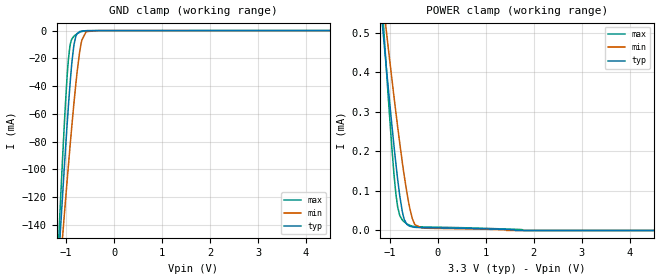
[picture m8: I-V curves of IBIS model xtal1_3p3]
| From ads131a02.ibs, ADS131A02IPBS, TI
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|   xtal1_3p3 Model
[Model]   xtal1_3p3
Model_type   Input
Vinl = 0.66
Vinh = 2.64
|   typ   min   max
|   (nom PVT)   (fast PVT)   (slow PVT)
C_comp   1.078e-12   1.069e-12   1.087e-12
| Where nom  PVT is Nominal Process, 3.3V, 27C
|   Fast PVT is Strong Process,  3.6V, -40C
|   Slow PVT is Weak Process,   3V, 125C
[Voltage Range]   3.3   3   3.6
|Junction Temperature
[Temperature Range]   27   125   -40
[Power Clamp Reference]   3.3   3   3.6
[GND Clamp Reference]   0   0   0
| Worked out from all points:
|   GND clamp passes 1 mA (typ) near -0.73 V on its own axis
[GND Clamp]
|   Voltage   I(typ)   I(min)   I(max)
-3.3V     -1.499A    -1.18A     -1.891A
-1.197V   -189.5mA   -202.3mA   -182.1mA
-1.115V   -141.8mA   -166.2mA   -121mA
-1.076V   -119.8mA   -149.3mA   -93.22mA
-985.2mV  -70.78mA   -110.8mA   -36.03mA
-924mV    -41.03mA   -85.7mA    -12.05mA
-838.2mV  -10.61mA   -52.65mA   -4.091mA
-720mV    -770.1uA   -15.88mA   -1.284mA
-672mV    -327.5uA   -6.863mA   -646.3uA
-582mV    -63.44uA   -776.3uA   -118.6uA
-330mV    -7.272uA   -6.598uA   -9.049uA
6.6V      0A         0A         0A
[POWER Clamp]
|   Voltage   I(typ)   I(min)   I(max)
-3.3V     3.499mA    3.018mA    4.843mA
-1.188V   562uA      627.7uA    621.7uA
-1.061V   395.7uA    491.1uA    385.6uA
-917.4mV  217.9uA    341.7uA    146.7uA
-873.6mV  167.9uA    297.7uA    91.33uA
-837.6mV  129.5uA    262.3uA    59.51uA
-792mV    86.18uA    218.9uA    37.33uA
-726mV    39.42uA    159.8uA    24.61uA
-597.3mV  11.41uA    63.63uA    13.78uA
-480mV    7.991uA    14.81uA    9.811uA
-330mV    7.19uA     5.948uA    8.994uA
6.6V      0A         0A         0A
